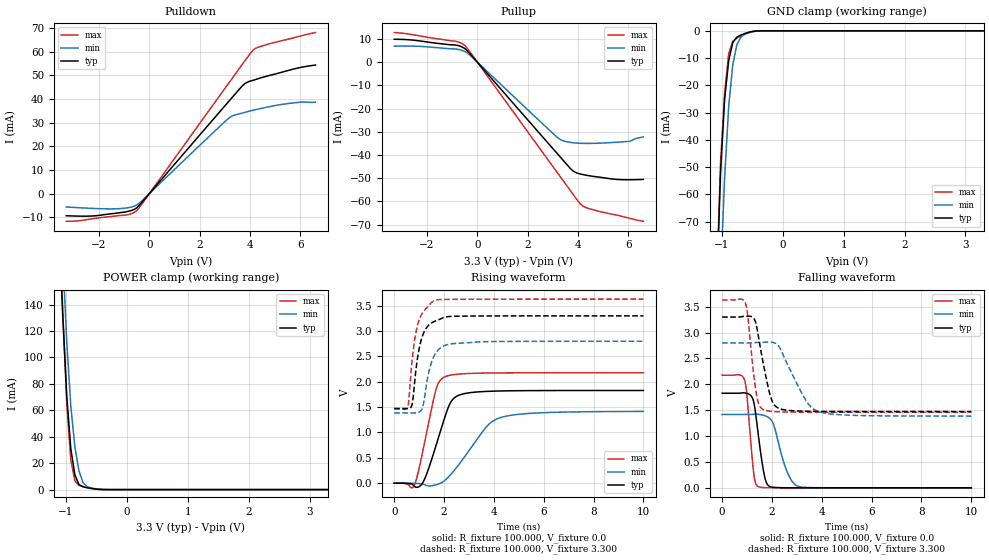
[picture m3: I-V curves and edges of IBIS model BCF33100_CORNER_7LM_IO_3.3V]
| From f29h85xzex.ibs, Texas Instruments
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|BCF33100_CORNER_7LM_IO_3.3V;
|   Model BCF33100_CORNER_7LM_IO_3.3V
[Model]   BCF33100_CORNER_7LM_IO_3.3V
Model_type   I/O
Polarity   Non-Inverting
Enable   Active-Low
Vinl =   0.800V
Vinh =   2.000V
Vmeas =  1.650V
Cref =   15.000pF
Vref =   0.0V
|   typ   min   max
C_comp   0.836pF   0.827pF   0.864pF
[Model Spec]
Vinh   2.000V   2.000V   2.000V
Vinl   0.800V   0.800V   0.800V
[Temperature Range]   25   155   -40
[Voltage Range]   3.300V   2.800V   3.630V
[Pullup Reference]   3.300V   2.800V   3.630V
[Pulldown Reference]   0.0V   0.0V   0.0V
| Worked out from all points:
|   slope of the pulldown table from 0 to 0.495 V, typ, clamps not added: 80.6 ohm
|   slope of the pullup table from 0 to 0.495 V, typ, clamps not added: 80.4 ohm
|   GND clamp passes 1 mA (typ) near -0.62 V on its own axis
|   POWER clamp passes 1 mA (typ) near -0.60 V on its own axis
|   rising waveform, R_fixture 100.000, V_fixture 0.0: 20-80 % time 711ps typ, 1.28ns min, 558ps max; typ from 0 V to 1.83 V
|   rising waveform, R_fixture 100.000, V_fixture 3.300: 20-80 % time 369ps typ, 399ps min, 359ps max; typ from 1.47 V to 3.3 V
|   falling waveform, R_fixture 100.000, V_fixture 0.0: 20-80 % time 310ps typ, 509ps min, 230ps max; typ from 1.83 V to 0 V
|   falling waveform, R_fixture 100.000, V_fixture 3.300: 20-80 % time 447ps typ, 892ps min, 292ps max; typ from 3.3 V to 1.47 V
[Pulldown]
|Voltage   I(typ)   I(min)   I(max)
-3.3V     -9.334mA   -5.624mA   -11.69mA
-2V       -9.188mA   -6.341mA   -10.22mA
-900mV    -7.614mA   -6.047mA   -8.971mA
-500mV    -5.98mA    -4.793mA   -7.12mA
3.1V      38.31mA    31.41mA    45.89mA
3.3V      40.76mA    32.85mA    48.84mA
3.7V      45.61mA    34.05mA    54.72mA
3.9V      47.13mA    34.65mA    57.66mA
4.1V      47.84mA    35.19mA    60.42mA
4.4V      48.85mA    35.91mA    62.15mA
5.5V      52.01mA    38.06mA    65.22mA
6.6V      54.34mA    38.67mA    68.07mA
[Pullup]
|Voltage   I(typ)   I(min)   I(max)
-3.3V     9.804mA    6.83mA     12.69mA
-2.3V     9.109mA    6.76mA     11.29mA
-900mV    7.366mA    5.643mA    9.036mA
-500mV    5.862mA    4.571mA    7.182mA
-300mV    3.729mA    3.062mA    4.5mA
3.2V      -39.67mA   -32.61mA   -47.88mA
3.4V      -42.14mA   -33.84mA   -50.87mA
3.8V      -46.84mA   -34.73mA   -56.83mA
4.1V      -48.21mA   -34.98mA   -61.12mA
4.4V      -48.86mA   -35.03mA   -62.96mA
6V        -50.67mA   -34.17mA   -67.1mA
6.6V      -50.52mA   -32.25mA   -68.55mA
[GND_clamp]
|Voltage   I(typ)   I(min)   I(max)
-3.3V     -2.491A    -2.028A    -3.569A
-1.089V   -97.28mA   -133.9mA   -96.44mA
-1.022V   -52.52mA   -90.69mA   -48.49mA
-955mV    -25.27mA   -54.25mA   -23.16mA
-888mV    -10.96mA   -27.87mA   -8.421mA
-821mV    -4.349mA   -12.46mA   -3.852mA
-754mV    -2.344mA   -5.125mA   -2.667mA
-687mV    -1.54mA    -2.273mA   -1.891mA
-620mV    -963.6uA   -1.185mA   -1.213mA
-553mV    -497.4uA   -634.4uA   -645.1uA
-352mV    -4.814uA   -27.17uA   -5.281uA
3.3V      0A         0A         0A
[POWER_clamp]
|Voltage   I(typ)   I(min)   I(max)
-3.3V     3.245A     3.678A     3.62A
-1.122V   207.3mA    257.6mA    223.8mA
-1.055V   132.9mA    178.5mA    137.2mA
-988mV    71.14mA    111.9mA    65.33mA
-921mV    30.87mA    63.02mA    22.54mA
-854mV    11.11mA    32.11mA    6.548mA
-787mV    3.796mA    14.03mA    3.209mA
-720mV    2.107mA    5.215mA    2.297mA
-653mV    1.419mA    2.207mA    1.575mA
-452mV    169.6uA    361.1uA    128.2uA
3.3V      0A         0A         0A
[Ramp]
| variable   typ   min   max
dV/dt_r   1.097/0.711n   0.850/1.279n   1.306/0.558n
dV/dt_f   1.095/0.446n   0.848/0.893n   1.301/0.292n
R_load = 100.000
[Rising Waveform]
R_fixture= 100.000
V_fixture= 0.0
V_fixture_min= 0.0
V_fixture_max= 0.0
|time   V(typ)   V(min)   V(max)
0s        4.81uV     4.52uV     8.31uV
812ps     -63.94mV   -2.81mV    -33.61mV
1.177ns   37.24mV    -21.67mV   700.5mV
1.666ns   723.8mV    -34.59mV   1.828V
2.043ns   1.316V     59.69mV    2.1V
2.285ns   1.609V     178.3mV    2.133V
2.555ns   1.726V     341.8mV    2.15V
3.664ns   1.809V     1.09V      2.172V
4.254ns   1.818V     1.291V     2.175V
10ns      1.828V     1.416V     2.177V
[Rising Waveform]
R_fixture= 100.000
V_fixture= 3.300
V_fixture_min= 2.800
V_fixture_max= 3.630
|time   V(typ)   V(min)   V(max)
0s        1.474V     1.385V     1.462V
547ps     1.472V     1.385V     1.505V
706ps     1.53V      1.384V     2.357V
808ps     1.93V      1.385V     2.787V
931ps     2.454V     1.392V     3.101V
1.078ns   2.815V     1.432V     3.308V
1.398ns   3.124V     2.208V     3.508V
1.608ns   3.189V     2.516V     3.602V
2.508ns   3.293V     2.758V     3.626V
10ns      3.3V       2.8V       3.63V
[Falling Waveform]
R_fixture= 100.000
V_fixture= 0.0
V_fixture_min= 0.0
V_fixture_max= 0.0
|time   V(typ)   V(min)   V(max)
0s        1.828V     1.418V     2.177V
900ps     1.834V     1.418V     2.08V
978ps     1.827V     1.418V     1.868V
1.274ns   1.648V     1.421V     258.1mV
1.456ns   1.009V     1.42V      23.67mV
1.826ns   60.08mV    1.37V      2.887mV
2.08ns    9.597mV    1.204V     1.491mV
2.636ns   1.963mV    279.2mV    608.5uV
3.081ns   1.047mV    24.59mV    309.3uV
10ns      2.111uV    96.61uV    1.637uV
[Falling Waveform]
R_fixture= 100.000
V_fixture= 3.300
V_fixture_min= 2.800
V_fixture_max= 3.630
|time   V(typ)   V(min)   V(max)
0s        3.3V       2.8V       3.63V
947ps     3.315V     2.8V       3.55V
1.227ns   3.295V     2.801V     2.369V
1.387ns   3.114V     2.809V     1.778V
1.692ns   2.303V     2.814V     1.504V
1.962ns   1.735V     2.814V     1.477V
2.16ns    1.57V      2.787V     1.471V
3.374ns   1.48V      1.68V      1.462V
3.834ns   1.477V     1.482V     1.462V
10ns      1.474V     1.385V     1.462V
